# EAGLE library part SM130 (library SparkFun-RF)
SonMicro SMB130 - 13.56 MHz RFID Mifare Read/Write Module The SMB130 is a 28 pin DIP module that includes all necessary components for a 13.56 MHz RFID MIFARE®, aside from a PCB antenna. SparkFun Products RFID Module - SM130 MIFARE® (13.56 MHz) (SEN-10126)
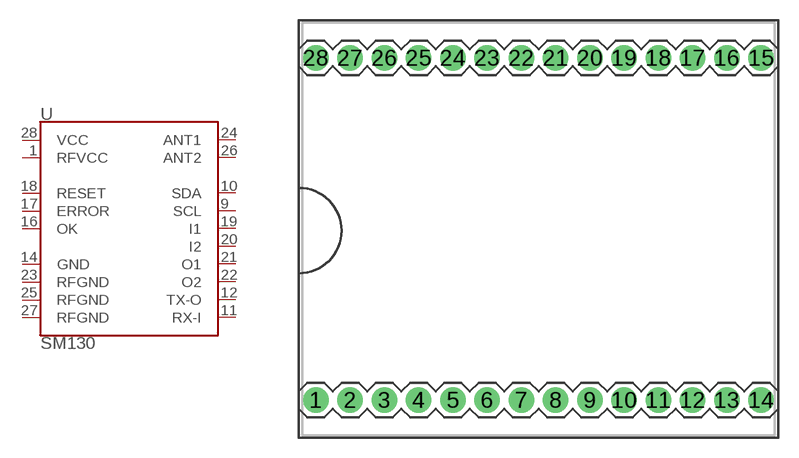
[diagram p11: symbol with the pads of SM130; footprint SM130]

Designator prefix U

## SM130 (PROD_ID: LPA-12905)  [SM130]
1  RFVCC
9  SCL
10  SDA
11  RX-I
12  TX-O
14  GND
16  OK
17  ERROR
18  RESET
19  I1
20  I2
21  O1
22  O2
23  RFGND
24  ANT1
25  RFGND
26  ANT2
27  RFGND
28  VCC

## Footprint SM130 (pad centres in mm)
SM130 13.56 MHz RFID Mifare(R) R/W Module 30-pin DIL with 100mil spacing between headers Datasheet
drill 1.016 pad 1.88: 1 -17.78,-12.7; 2 -15.24,-12.7; 3 -12.7,-12.7; 4 -10.16,-12.7; 5 -7.62,-12.7; 6 -5.08,-12.7; 7 -2.54,-12.7; 8 0,-12.7; 9 2.54,-12.7; 10 5.08,-12.7; 11 7.62,-12.7; 12 10.16,-12.7; 13 12.7,-12.7; 14 15.24,-12.7; 15 15.24,12.7; 16 12.7,12.7; 17 10.16,12.7; 18 7.62,12.7; 19 5.08,12.7; 20 2.54,12.7; 21 0,12.7; 22 -2.54,12.7; 23 -5.08,12.7; 24 -7.62,12.7; 25 -10.16,12.7; 26 -12.7,12.7; 27 -15.24,12.7; 28 -17.78,12.7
